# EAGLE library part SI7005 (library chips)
Si7005 Digital I2C Humidity and Temperature Sensor
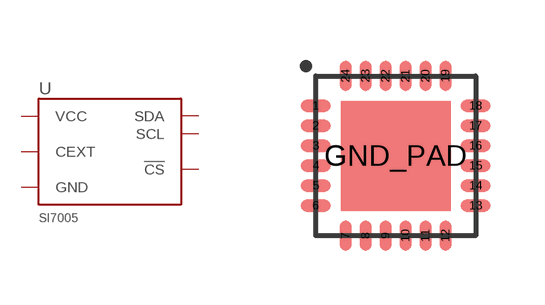
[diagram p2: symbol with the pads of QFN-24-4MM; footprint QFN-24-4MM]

Designator prefix U

## SI7005 (DIGIKEY: 336-2332-1-ND)  [QFN-24-4MM]
1  GND
3  SCL
4  SDA
8  GND
9  VCC
10  CEXT
11  GND
15  !CS
19  GND
GND_PAD  GND

## Footprint QFN-24-4MM (pad centres in mm)
4mm x 4mm QFN-24
smd 0.75 x 0.3: 1 -2,1.25; 2 -2,0.75; 3 -2,0.25; 4 -2,-0.25; 5 -2,-0.75; 6 -2,-1.25; 13 2,-1.25; 14 2,-0.75; 15 2,-0.25; 16 2,0.25; 17 2,0.75; 18 2,1.25
smd 0.3 x 0.75: 7 -1.25,-2; 8 -0.75,-2; 9 -0.25,-2; 10 0.25,-2; 11 0.75,-2; 12 1.25,-2; 19 1.25,2; 20 0.75,2; 21 0.25,2; 22 -0.25,2; 23 -0.75,2; 24 -1.25,2
smd 2.75 x 2.75: GND_PAD 0,0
